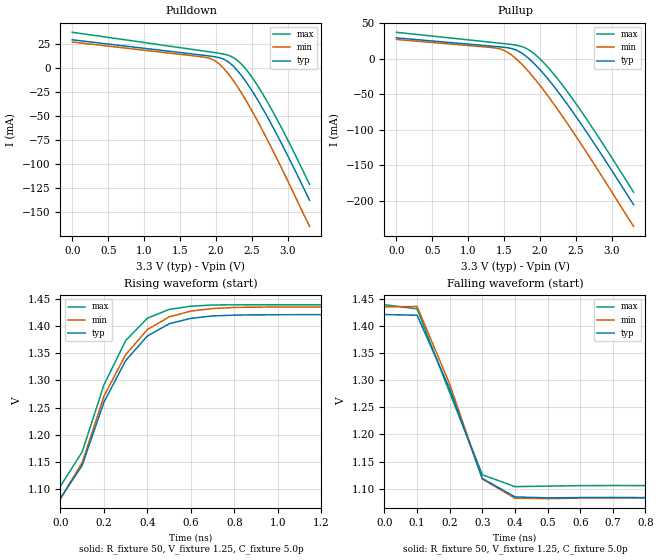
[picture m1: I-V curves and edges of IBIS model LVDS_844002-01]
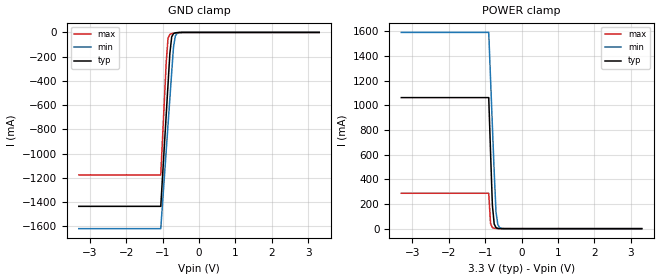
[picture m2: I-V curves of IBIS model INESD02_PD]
|   This file is an IBIS representation of the   |
|   Integrated Device Technology, Inc.   |
|   ICS844002-01   |
[IBIS Ver]   4.0
[File name]   844002-01_3v3.ibs
[File Rev]   1.0
[Date]   Sep 7 2007  | Last modified
|   Sep 7 2007  | Generated
[Source] Originated at Integrated Device Technology, Inc.
[Disclaimer]
IDT hereby grants the user of this IBIS model a non-exclusive,
nontransferable license to use this IBIS model under the following terms.
Before using this IBIS model, the user should read this license.
If the user does not accept these terms,  the IBIS model should be
returned to IDT within 30 days.
   The user is granted this license only to use the IBIS model and
is not granted rights to sell, load, rent, lease or license the IBIS
model in whole or in part, or in modified form to anyone other than
user. User may modify the IBIS model to suit its specific
applications but rights to derivative works and such modifications
shall belong to IDT.
   This IBIS model is provided on an "AS IS" basis and IDT makes
absolutely no warranty with respect to the information contained
herein. IDT DISCLAIMS AND CUSTOMER WAIVES ALL WARRANTIES, EXPRESS
OR IMPLIED, INCLUDING WARRANTIES OF MERCHANTABILITY OR FITNESS FOR
A PARTICULAR PURPOSE. The entire risk as to quality and performance
is with the Customer. ACCORDINGLY, IN NO EVENT SHALL THE COMPANY BE
LIABLE FOR ANY DAMAGES, WHETHER IN CONTRACT OR TORT,INCLUDING ANY
LOST PROFITS OR OTHER INCIDENTAL, CONSEQUENTIAL, EXEMPLARY, OR
PUNITIVE DAMAGES ARISING OUT OF THE USE OR APPLICATION OF THE IBIS
model provided in this package. Further, IDT reserves the right to
make changes without notice to any product herein to improve
reliability, function, or design. IDT does not convey any license
under patent rights or any other intellectual property rights,
including those of third parties.
   IDT is not obligated to provide maintenance or support
for the licensed IBIS model.
[Copyright]   Copyright 2007 by Integrated Device Technology, Inc.
[Component]   ICS844002AG-01
[Manufacturer] Integrated Device Technology, Inc.
[Package]
|TSSOP 20 Lead
|   typ   min   max
R_pkg   51.85m   41.1m   62.6m
L_pkg   1.568nH   0.734nH   2.401nH
C_pkg   0.221pF   0.068pF   0.373pF
[Pin] signal_name  model_name   R_pin   L_pin   C_pin
|1   nc   62.6m   2.401n   0.373p
2   VDDO   POWER   57.23m   1.985n   0.297p
3   Q0   LVDS_844002-01   51.85m   1.568n   0.221p
4   nQ0   LVDS_844002-01   46.78m   1.151n   0.145p
5   MR   INESD02_PD   41.1m   0.734n   0.068p
6   nPLL_SEL   INESD02_PD   41.1m   0.734n   0.068p
|7   nc   46.78m   1.151n   0.145p
8   VDDA   POWER   51.85m   1.568n   0.221p
9   F_SEL0   INESD02_PD   57.23m   1.985n   0.297p
10   VDD   POWER   62.6m   2.401n   0.373p
11   F_SEL1   INESD02_PD   62.6m   2.401n   0.373p
|12  XTAL_OUT   57.23m   1.985n   0.297p
|13  XTAL_IN   51.85m   1.568n   0.221p
14   REF_CLK   INESD02_PD   46.78m   1.151n   0.145p
15   nXTAL_SEL   INESD02_PD   41.1m   0.734n   0.068p
16   VDD   POWER   41.1m   0.734n   0.068p
17   GND   GND   46.78m   1.151n   0.145p
18   nQ1   LVDS_844002-01   51.85m   1.568n   0.221p
19   Q1   LVDS_844002-01   57.23m   1.985n   0.297p
20   VDDO   POWER   62.6m   2.401n   0.373p
| Models and submodels in the file (2): LVDS_844002-01 (Output_ECL), INESD02_PD (Input)
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[Model]   LVDS_844002-01
|onlvds01_lvds03_vrlvds06-abiasoff01_3V3
Model_type   Output_ECL
Polarity   Non-Inverting
|   typ   min   max
C_comp   2pF   1.5pF   2.5pF
Vmeas = 1.25V
Rref = 50
Vref = 1.25V
|   typ   min   max
[Voltage range]   3.3V   3.135V   3.465V
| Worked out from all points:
|   rising waveform, R_fixture 50, V_fixture 1.25, C_fixture 5.0p: 20-80 % time 231ps typ, 234ps min, 196ps max; typ from 1.08 V to 1.42 V
|   falling waveform, R_fixture 50, V_fixture 1.25, C_fixture 5.0p: 20-80 % time 132ps typ, 130ps min, 131ps max; typ from 1.42 V to 1.08 V
[pulldown]
|Voltage   I (typ)   I (min)   I (max)
0V        29.08mA    26.8mA     36.89mA
1.8V      13.22mA    11.37mA    17.73mA
1.9V      12.32mA    10.03mA    16.66mA
2V        11.24mA    6.613mA    15.58mA
2.15V     7.191mA    -4.325mA   13.43mA
2.25V     965.3uA    -14.33mA   10.19mA
2.35V     -7.741mA   -25.77mA   4.035mA
2.5V      -23.89mA   -44.84mA   -9.868mA
2.65V     -42.52mA   -65.56mA   -27.29mA
2.85V     -69.92mA   -94.93mA   -53.84mA
3.05V     -99.22mA   -125.7mA   -82.8mA
3.3V      -137.5mA   -164.6mA   -121mA
[pullup]
|Voltage   I (typ)   I (min)   I (max)
0V        29.08mA    26.8mA     36.89mA
1.35V     17.18mA    15.14mA    22.52mA
1.5V      15.75mA    11.38mA    20.91mA
1.6V      14.13mA    5.181mA    19.77mA
1.75V     7.285mA    -8.508mA   16.68mA
1.9V      -5.36mA    -25.52mA   8.171mA
2.05V     -21.61mA   -44.7mA    -5.816mA
2.2V      -40.2mA    -65.36mA   -23.15mA
2.4V      -67.42mA   -94.5mA    -49.51mA
2.65V     -104mA     -132.6mA   -85.74mA
2.95V     -150.1mA   -180mA     -132mA
3.3V      -205.5mA   -235.9mA   -187.9mA
[Ramp]
|   typ   min   max
dV/dt_r   0.24/0.3n   0.24/0.35n   0.24/0.25n
dV/dt_f   0.24/0.3n   0.24/0.35n   0.24/0.25n
[Rising Waveform]
R_fixture = 50
V_fixture = 1.25
V_fixture_max = 1.28
V_fixture_min = 1.22
C_fixture = 5.0p
| Time   typ   min   max
0s        1.083V     1.083V     1.106V
100ps     1.144V     1.149V     1.169V
200ps     1.26V      1.271V     1.292V
300ps     1.336V     1.347V     1.373V
400ps     1.381V     1.393V     1.414V
500ps     1.404V     1.416V     1.43V
600ps     1.414V     1.427V     1.436V
800ps     1.42V      1.434V     1.438V
1ns       1.42V      1.435V     1.439V
5ns       1.421V     1.435V     1.439V
[Falling Waveform]
R_fixture = 50
V_fixture = 1.25
V_fixture_max = 1.28
V_fixture_min = 1.22
C_fixture = 5.0p
| Time   typ   min   max
0s        1.421V     1.435V     1.439V
100ps     1.419V     1.435V     1.431V
200ps     1.284V     1.292V     1.277V
300ps     1.119V     1.118V     1.126V
400ps     1.085V     1.083V     1.104V
500ps     1.083V     1.082V     1.105V
700ps     1.084V     1.083V     1.106V
5ns       1.083V     1.083V     1.106V
[Model]   INESD02_PD
Model_type   Input
Polarity   Non-Inverting
Vinl = 0.80V
Vinh = 2.0V
|   typ   min   max
C_comp   2pF   1.5pF   2.5pF
|   typ   min   max
[Voltage range]  3.3V   3.15V   3.45V
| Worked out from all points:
|   GND clamp passes 1 mA (typ) near -0.56 V on its own axis
|   POWER clamp passes 1 mA (typ) near -0.61 V on its own axis
[GND_clamp]
|Voltage   I(typ)   I(min)   I(max)
-3.3V     -1.436A    -1.62A     -1.176A
-1.05V    -1.436A    -1.62A     -1.176A
-900mV    -678.5mA   -975.1mA   -244mA
-850mV    -426.1mA   -760.1mA   -46.85mA
-800mV    -173.9mA   -545.4mA   -16.11mA
-750mV    -36.96mA   -330.7mA   -9.916mA
-700mV    -9.696mA   -120.2mA   -7.056mA
-650mV    -3.545mA   -29.7mA    -4.857mA
-600mV    -1.629mA   -7.52mA    -3.049mA
-400mV    -52.81uA   -52.52uA   -108.7uA
3.3V      71.13uA    77.43uA    62.11uA
[POWER_clamp]
|Voltage   I(typ)   I(min)   I(max)
-3.3V     1.063A     1.593A     287.3mA
-900mV    1.063A     1.593A     287.3mA
-850mV    620.5mA    1.215A     41.84mA
-800mV    191.6mA    837.5mA    8.757mA
-750mV    37.76mA    460.2mA    3.328mA
-700mV    8.104mA    133.8mA    1.728mA
-650mV    2.076mA    32.66mA    905.3uA
-600mV    678.1uA    8.083mA    443.8uA
-450mV    104.2uA    213.3uA    89.09uA
3.3V      -3.041nA   -3.986uA   0A
